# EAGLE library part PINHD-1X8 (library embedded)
PIN HEADER
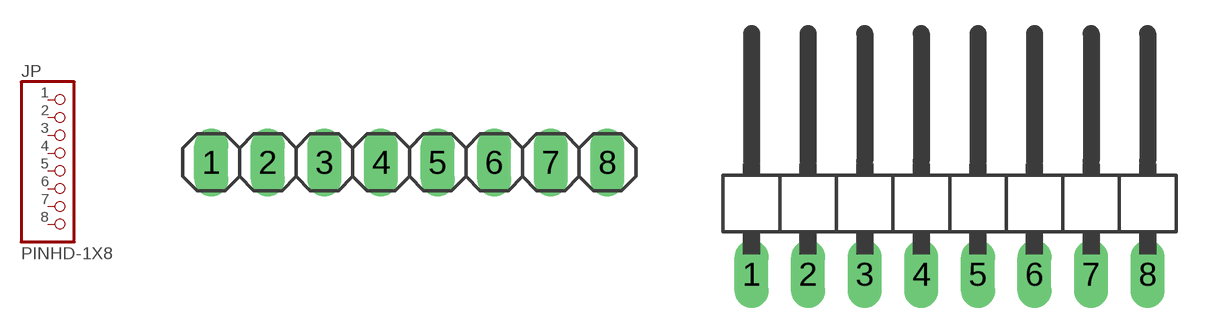
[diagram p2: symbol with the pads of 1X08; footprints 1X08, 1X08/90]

Designator prefix JP

## PINHD-1X8 (ANGLE: Straight; PACKAGE: Pin Header; PITCH: 2.54mm; POS: 8; ROWS: 1)  [1X08]
1  1  pas
2  2  pas
3  3  pas
4  4  pas
5  5  pas
6  6  pas
7  7  pas
8  8  pas

## PINHD-1X8/90 (ANGLE: 90; PACKAGE: Pin Header; PITCH: 2.54mm; POS: 8; ROWS: 1)  [1X08/90]
Pads as for 1X08

## Footprint 1X08 (pad centres in mm)
PIN HEADER
drill 1.016 long: 1 -8.89,0; 2 -6.35,0; 3 -3.81,0; 4 -1.27,0; 5 1.27,0; 6 3.81,0; 7 6.35,0; 8 8.89,0

## Footprint 1X08/90 (pad centres in mm)
PIN HEADER
drill 1.016 long: 1 -8.89,-3.81; 2 -6.35,-3.81; 3 -3.81,-3.81; 4 -1.27,-3.81; 5 1.27,-3.81; 6 3.81,-3.81; 7 6.35,-3.81; 8 8.89,-3.81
